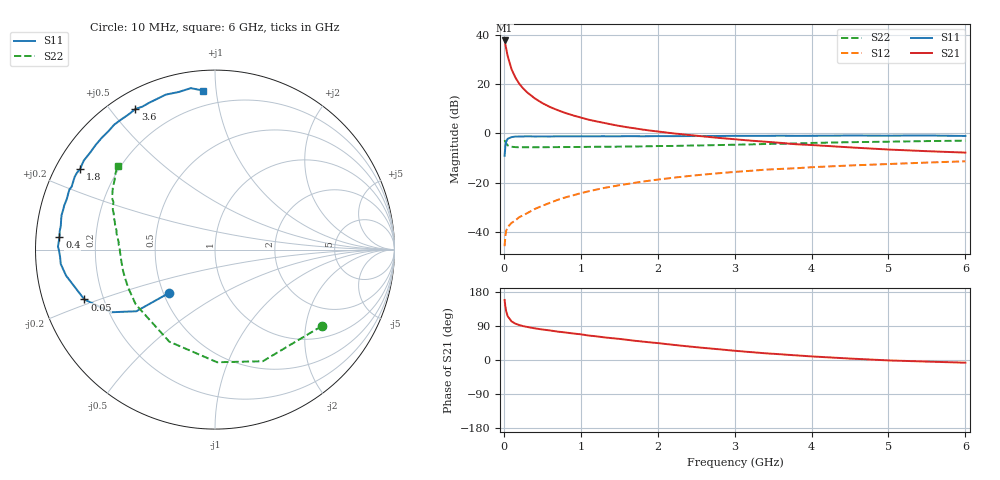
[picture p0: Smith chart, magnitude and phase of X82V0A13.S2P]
! SIEMENS Small Signal Semiconductors
! BFP136W
! Si NPN RF Bipolar Junction Transistor in SOT343
! VCE = 2 V  IC = 130 mA
! Common Emitter S-Parameters:  September  1994
# GHz  S  MA  R  50
!  f  S11  S21  S12  S22
! GHz  MAG  ANG  MAG  ANG  MAG  ANG  MAG  ANG
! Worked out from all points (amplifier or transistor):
!   40 points, 10 MHz to 6 GHz, reference 50 ohm
!   highest |S21| = 37.7 dB at 10 MHz (marker M1)
!   |S21| within 3 dB of that: start of sweep to 28.7 MHz
!   unconditionally stable (mu >= 1): 414.5 MHz to 2.938 GHz; 3.794204 GHz to 3.809963 GHz; 5.974912 GHz to end of sweep
!   at 200 MHz: K = 0.76, MSG = 27.0 dB, |S12| = -33.9 dB
!   at 1.5 GHz: K = 1.12, MAG = 9.9 dB, |S12| = -21.0 dB
!   at 6 GHz: K = 1.00, MAG = 1.4 dB, |S12| = -11.3 dB
!   S11 on the Smith chart (normalised r, x): 10 MHz: 0.53, -0.30; 50 MHz: 0.13, -0.18; 400 MHz: 0.07, +0.04; 1.8 GHz: 0.07, +0.27; 3.6 GHz: 0.07, +0.58; 6 GHz: 0.11, +0.92
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0.01  0.3527 -136.7  76.53 158.4  0.0052 65.9  0.7318 -35.6
0.02  0.5568 -141.9  64.09 141.0  0.0084 53.4  0.6767 -66.8
0.03  0.6758 -148.9  52.84 129.0  0.0106 47.9  0.6278 -88.9
0.05  0.7791 -159.1  36.82 115.5  0.0127 38.6  0.5726 -116.4
0.1  0.8425 -170.1  20.04 101.9  0.0154 37.5  0.5369 -145.3
0.15  0.8631 -174.7  13.58 95.9  0.0173 41.9  0.5283 -156.6
0.2  0.8642 -177.4  10.18 92.2  0.0201 45.5  0.5255 -162.6
0.25  0.8693 -179.7  8.202 89.4  0.022 49.2  0.526 -166.5
0.3  0.8751 178.9  6.858 87.4  0.0241 51.8  0.525 -169.1
0.4  0.8694 175.5  5.161 83.6  0.0294 56.1  0.5257 -172.6
0.5  0.8712 173.2  4.116 80.5  0.0342 59.4  0.5265 -175.0
0.6  0.8693 171.2  3.435 78.0  0.0393 61.0  0.5273 -176.6
0.7  0.8737 168.8  2.961 74.9  0.0451 62.9  0.5287 -177.8
0.9  0.8745 165.5  2.321 70.0  0.0557 63.4  0.5308 179.7
1.1  0.8724 161.3  1.901 64.6  0.0671 63.4  0.5341 178.1
1.8  0.8749 149.2  1.201 48.7  0.1055 59.6  0.5465 172.5
2.2  0.8808 142.5  1.004 40.1  0.1265 56.1  0.5581 169.4
3.2  0.8936 125.6  0.717 21.0  0.1746 46.0  0.5991 160.4
3.6  0.9002 119.5  0.644 15.1  0.1911 41.9  0.6179 156.9
4.5  0.906 107.6  0.522 3.8  0.2243 33.2  0.6647 148.9
5.5  0.9095 98.5  0.437 -4.2  0.2568 25.1  0.6998 142.3
6  0.8885 94.3  0.409 -7.1  0.2728 20.7  0.713 139.4
